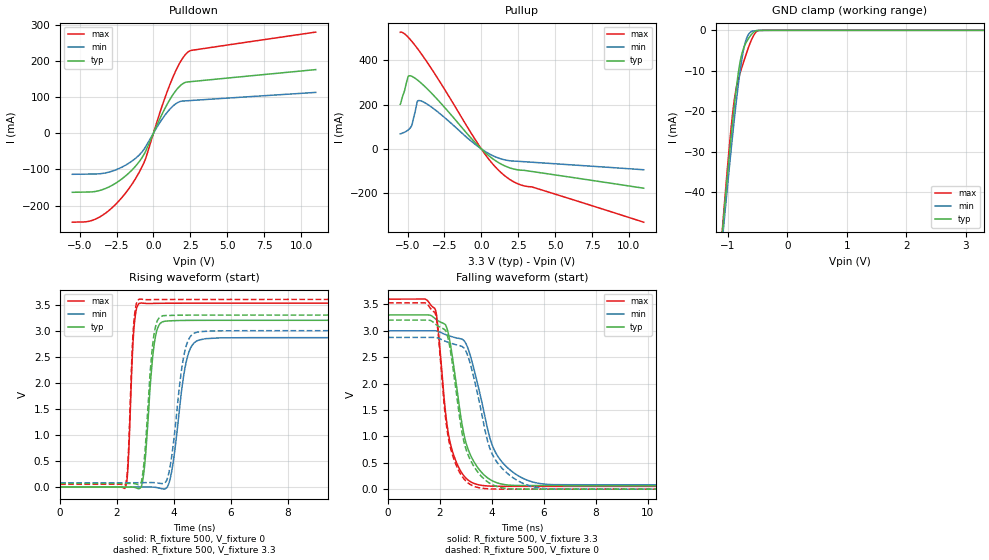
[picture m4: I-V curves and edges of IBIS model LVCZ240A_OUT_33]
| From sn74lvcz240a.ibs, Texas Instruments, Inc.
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[Model]   LVCZ240A_OUT_33
Model_type  3-state
Enable   Active-Low
Vref =   0
Rref =   500
Cref =   30p
Vmeas =   1.65
| variable   typ   min   max
C_comp   4.46pF   NA   NA
| C_pullup   6.24pF   4.12pF   7.61pF
| C_pulldown   5.55pF   4.87pF   6.86pF
| C_tri-state   4.46pF   3.72pF   5.61pF
[Temperature Range]   40   100   -40
| Ambient temperature   25   85   -40
[Voltage range]   3.3   3   3.6
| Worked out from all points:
|   slope of the pulldown table from 0 to 0.495 V, typ, clamps not added: 11 ohm
|   slope of the pullup table from 0 to 0.495 V, typ, clamps not added: 16.5 ohm
|   GND clamp passes 1 mA (typ) near -0.60 V on its own axis
|   rising waveform, R_fixture 500, V_fixture 0: 20-80 % time 260ps typ, 393ps min, 153ps max; typ from 0 V to 3.2 V
|   falling waveform, R_fixture 500, V_fixture 3.3: 20-80 % time 684ps typ, 943ps min, 498ps max; typ from 3.3 V to 0.068 V
|   rising waveform, R_fixture 500, V_fixture 3.3: 20-80 % time 251ps typ, 375ps min, 149ps max; typ from 0.068 V to 3.3 V
|   falling waveform, R_fixture 500, V_fixture 0: 20-80 % time 669ps typ, 902ps min, 493ps max; typ from 3.2 V to 0 V
[GND Clamp]
| LVCZ240A_OUT_33
|   Voltage   I(typ)   I(min)   I(max)
-5.5V     -895mA     -842.7mA   -981.5mA
-1.095V   -50.24mA   -52.15mA   -49.52mA
-1.065V   -45.25mA   -47.46mA   -44.06mA
-960mV    -28.49mA   -31.6mA    -26.23mA
-915mV    -21.85mA   -25.17mA   -19.84mA
-880mV    -17.05mA   -20.4mA    -15.99mA
-805mV    -8.678mA   -11.19mA   -11.09mA
-740mV    -4.594mA   -5.061mA   -8.004mA
-685mV    -2.785mA   -1.952mA   -5.541mA
-620mV    -1.319mA   -449.7uA   -2.918mA
-480mV    -13.06uA   -50.96uA   -17.85uA
3.3V      18.67pA    44.83nA    -1.752nA
[Pulldown]
| LVCZ240A_OUT_33
|   Voltage   I(typ)   I(min)   I(max)
-5.5V     -163.3mA   -113.6mA   -245.8mA
-4.38V    -162.4mA   -112.9mA   -243.4mA
-3.505V   -156.6mA   -111.5mA   -228mA
-2.485V   -136.2mA   -100.2mA   -193.3mA
-1.495V   -103.2mA   -78.17mA   -143.2mA
-935mV    -76.94mA   -58.96mA   -105.3mA
-560mV    -52.46mA   -39.21mA   -73.23mA
465mV     42.5mA     31.24mA    60.21mA
1.14V     94.74mA    67.49mA    136.9mA
1.79V     130mA      87.2mA     194.4mA
2.345V    141.5mA    89.67mA    224.1mA
11V       175.5mA    112.6mA    279.1mA
[Pullup]
| LVCZ240A_OUT_33
|   Voltage   I(typ)   I(min)   I(max)
-5.5V     201.7mA    68.1mA     526.6mA
-4.95V    328.4mA    86.38mA    503.4mA
-4.7V     327.4mA    110.1mA    484.5mA
-4.345V   311.9mA    214mA      454.3mA
-4.145V   300.9mA    217.8mA    436.2mA
-3.06V    229.3mA    172.8mA    329mA
85mV      -5.565mA   -3.915mA   -8.347mA
865mV     -48.79mA   -33.02mA   -75.08mA
1.64V     -78.02mA   -49.97mA   -124mA
2.675V    -95.71mA   -56.52mA   -162.4mA
3.405V    -101.5mA   -59.75mA   -170.9mA
11V       -177.1mA   -93.79mA   -330.6mA
[Ramp]
| LVCZ240A_OUT_33
| variable   typ   min   max
dV/dt_r   1.94/2.72E-10   1.74/4.06E-10   2.13/1.56E-10
dV/dt_f   1.94/6.89E-10   1.75/9.46E-10   2.13/5.02E-10
R_load = 500
[Rising Waveform]
| LVCZ240A_OUT_33
R_fixture =   500
C_fixture =   0
L_fixture =   0
V_fixture =   0
V_fixture_min = 0
V_fixture_max = 0
|   Time   V(typ)   V(min)   V(max)
0s        171.1pV    2.972nV    26.69nV
2.29ns    -617.6uV   -445.7uV   -13.8mV
2.395ns   -190.1uV   -507.3uV   473.5mV
2.6ns     -4.09mV    -477.8uV   3.069V
2.85ns    -425.3uV   -388.4uV   3.532V
3.315ns   2.764V     -3.666mV   3.524V
3.705ns   3.184V     -31.84mV   3.526V
4.48ns    3.197V     2.503V     3.527V
5.12ns    3.199V     2.847V     3.527V
50ns      3.2V       2.866V     3.528V
[Falling Waveform]
| LVCZ240A_OUT_33
R_fixture =   500
C_fixture =   0
L_fixture =   0
V_fixture =   3.3
V_fixture_min = 3
V_fixture_max = 3.6
|   Time   V(typ)   V(min)   V(max)
0s        3.3V       3V         3.6V
1.805ns   3.235V     3.001V     3.419V
2.21ns    3.116V     2.929V     1.479V
2.475ns   2.52V      2.886V     727.4mV
2.965ns   949.7mV    2.788V     228.8mV
3.61ns    315mV      1.659V     72.02mV
3.97ns    171.1mV    897.1mV    57.74mV
4.355ns   99.31mV    537.7mV    54.17mV
6.15ns    67.95mV    90.19mV    53.03mV
50ns      67.71mV    82.34mV    52.81mV
[Rising Waveform]
| LVCZ240A_OUT_33
R_fixture =   500
C_fixture =   0
L_fixture =   0
V_fixture =   3.3
V_fixture_min = 3
V_fixture_max = 3.6
|   Time   V(typ)   V(min)   V(max)
0s        67.67mV    82.26mV    52.8mV
2.29ns    67.99mV    81.96mV    46.21mV
2.385ns   68.82mV    82.06mV    478.4mV
2.585ns   67.9mV     82.53mV    3.11V
2.785ns   49.7mV     83.18mV    3.606V
3.29ns    2.885V     85.22mV    3.596V
3.62ns    3.288V     64.84mV    3.599V
4.4ns     3.298V     2.639V     3.599V
4.925ns   3.299V     2.982V     3.6V
50ns      3.3V       3V         3.6V
[Falling Waveform]
| LVCZ240A_OUT_33
R_fixture =   500
C_fixture =   0
L_fixture =   0
V_fixture =   0
V_fixture_min = 0
V_fixture_max = 0
|   Time   V(typ)   V(min)   V(max)
0s        3.202V     2.874V     3.528V
1.805ns   3.136V     2.875V     3.343V
2.21ns    3.01V      2.801V     1.371V
2.465ns   2.425V     2.758V     674.4mV
2.93ns    887.5mV    2.67V      191.7mV
3.605ns   237.9mV    1.441V     19.05mV
3.91ns    114.6mV    790.6mV    5.996mV
4.31ns    34.34mV    440.7mV    1.509mV
6.12ns    262.7uV    7.063mV    229uV
50ns      32.83uV    74.05uV    10.83uV
